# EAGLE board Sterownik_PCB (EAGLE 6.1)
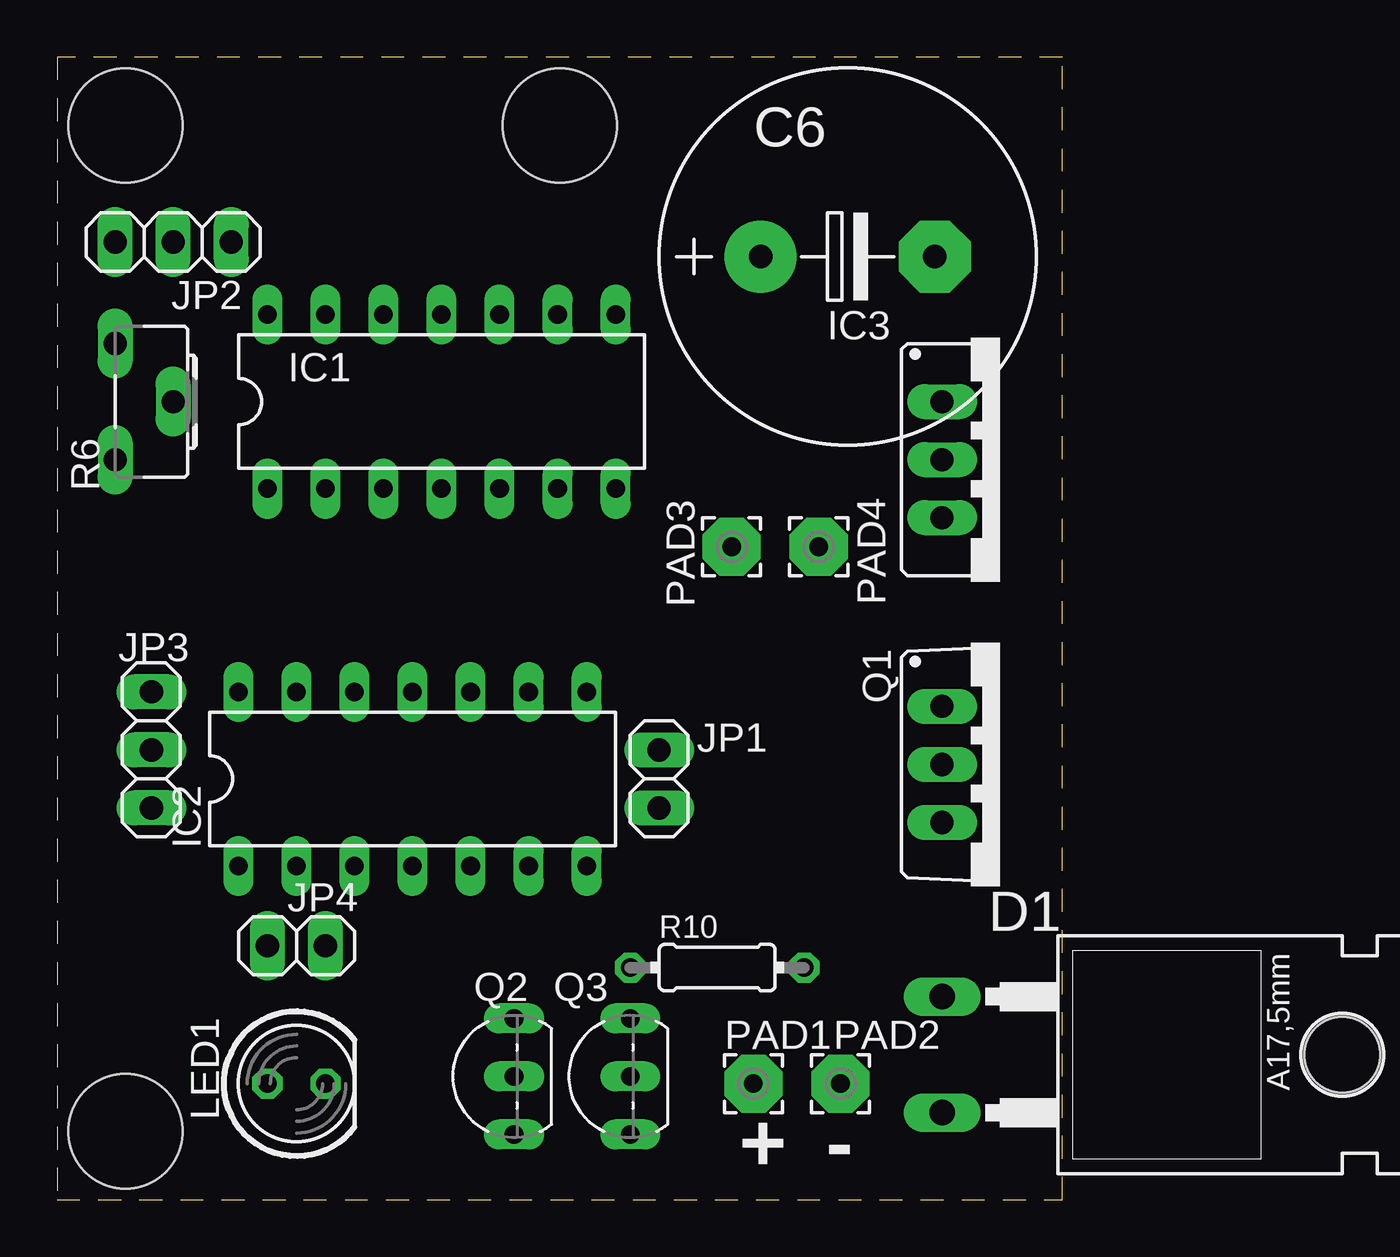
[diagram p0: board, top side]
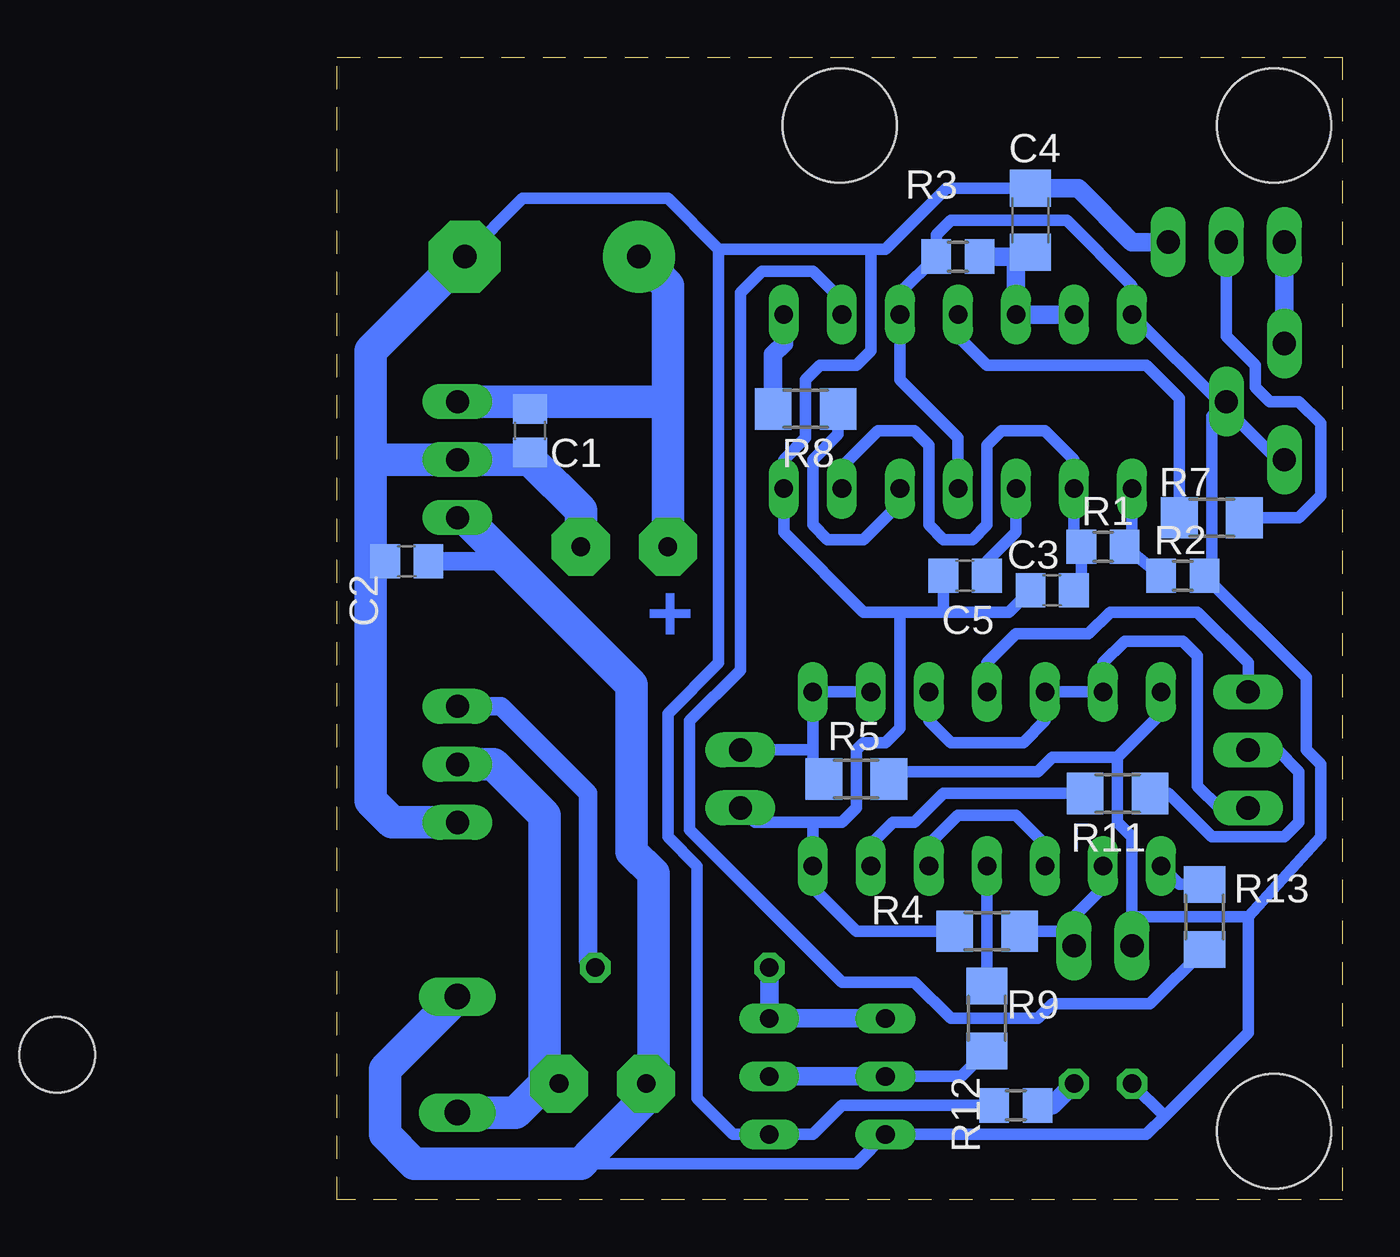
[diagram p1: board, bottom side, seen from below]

Size 44 x 50 mm. Coordinates in mm from the lower left corner, seen from the top.
Outline: 0,0 44,0 44,50 0,50 0,0
Copper layers (1*16): Top 0.035mm / dielectric 1.5mm / Bottom 0.035mm
Design rules: minimum track width 20mil, minimum drill 24mil, track to track 8mil, track to pad 8mil, pad to pad 8mil, via to via 8mil, smd to smd 8mil, copper to edge 10mil, drill to drill 8mil, minimum pad ring 10mil, minimum via ring 8mil, stop-mask expansion 4mil, vias tented up to drill 0mil, thermal gap 10mil
Holes 5 mm at 3,47 3,3 22,47

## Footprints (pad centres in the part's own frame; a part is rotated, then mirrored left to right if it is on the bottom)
C0805 = smd 1.3 x 1.5: 1 -0.95,0; 2 0.95,0
C1206 = smd 1.6 x 1.8: 1 -1.4,0; 2 1.4,0
E7,5-16 = drill 1.016 pad 3.15: + -3.81,0 | drill 1.016 pad 3.15 octagon: - 3.81,0
TO220AC = drill 1.118 long: A 2.54,-6.35; C -2.54,-6.35 | hole 3.302: 0,11.176
DIL14 = drill 0.813 long: 1 -7.62,-3.81; 2 -5.08,-3.81; 3 -2.54,-3.81; 4 0,-3.81; 5 2.54,-3.81; 6 5.08,-3.81; 7 7.62,-3.81; 8 7.62,3.81; 9 5.08,3.81; 10 2.54,3.81; 11 0,3.81; 12 -2.54,3.81; 13 -5.08,3.81; 14 -7.62,3.81
78XXS = drill 1.016 long: GND 0,-2.54; IN -2.54,-2.54; OUT 2.54,-2.54
1X02 = drill 1.016 long: 1 -1.27,0; 2 1.27,0
1X03 = drill 1.016 long: 1 -2.54,0; 2 0,0; 3 2.54,0
LED5MM = drill 0.813 octagon: A -1.27,0; K 1.27,0
2,54/0,8 = drill 0.813 pad 2.54 octagon: 1 0,0
TO220BV = drill 1.016 long: D 0,-2.54; G -2.54,-2.54; S 2.54,-2.54
TO92-EBC = drill 0.813 long: B 0,-1.27; C -2.54,-1.27; E 2.54,-1.27
R0805 = smd 1.3 x 1.5: 1 -0.95,0; 2 0.95,0
R1206 = smd 1.6 x 1.803: 1 -1.422,0; 2 1.422,0
CA6H = drill 1.016 long: A -2.54,0; E 2.54,0; S 0,2.54
0204/7 = drill 0.813 octagon: 1 -3.81,0; 2 3.81,0

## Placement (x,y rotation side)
C1  100n  [C0805]  35.56,33.66 270 bottom
C2  100n  [C0805]  40.96,27.94 180 bottom
C3  100n  [C0805]  12.7,26.67 180 bottom
C4  100n  [C1206]  13.65,42.86 90 bottom
C5  10n  [C0805]  16.51,27.3 180 bottom
C6  4700u  [E7,5-16]  34.61,41.27 0 top
D1  MBR1060  [TO220AC]  45.09,6.35 270 top
IC1  NE556N  [DIL14]  16.83,34.92 0 top
IC2  4093N  [DIL14]  15.56,18.41 0 top
IC3  78S12  [78XXS]  41.27,32.38 270 top
JP1  Switch  [1X02]  26.35,18.41 270 top
JP2  Obroty  [1X03]  5.08,41.91 0 top
JP3  Polaryzacja  [1X03]  4.13,19.68 90 top
JP4  Generator  [1X02]  10.48,11.11 0 top
LED1  G  [LED5MM]  10.48,5.08 0 top
PAD1  [2,54/0,8]  30.48,5.08 0 top
PAD2  [2,54/0,8]  34.29,5.08 0 top
PAD3  [2,54/0,8]  29.53,28.57 0 top
PAD4  [2,54/0,8]  33.34,28.57 0 top
Q1  IRF520  [TO220BV]  41.27,19.05 270 top
Q2  BC546B  [TO92-EBC]  18.73,5.4 90 top
Q3  BC558C  [TO92-EBC]  23.81,5.4 90 top
R1  10k  [R0805]  10.48,28.57 0 bottom
R2  4k7  [R0805]  6.99,27.3 0 bottom
R3  10k  [R0805]  16.83,41.27 180 bottom
R4  10k  [R1206]  15.56,11.75 0 bottom
R5  10k  [R1206]  21.27,18.41 0 bottom
R6  10k  [CA6H]  2.54,34.92 270 top
R7  0  [R1206]  5.71,29.84 180 bottom
R8  0  [R1206]  23.5,34.61 180 bottom
R9  10k  [R1206]  15.56,7.94 270 bottom
R10  33  [0204/7]  28.89,10.16 0 top
R11  0  [R1206]  9.84,17.78 180 bottom
R12  2k2  [R0805]  14.29,4.13 0 bottom
R13  0  [R1206]  6.03,12.38 90 bottom

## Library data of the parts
C1-C6 R1-R5 R7-R13 = rcl
D1 = diode
IC1 = linear
IC2 = 40xx
IC3 = v-reg
JP1-JP4 = pinhead
LED1 = led
PAD1-PAD4 = wirepad
Q1 = transistor-power
Q2 = transistor-npn
Q3 = transistor-pnp
R6 = pot

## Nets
+12V: C2.1 D1.C IC1.4 IC1.10 IC1.14 IC2.14 IC3.OUT JP4.1 LED1.A PAD1.1 Q2.C R2.2 R3.2 R5.2 R6.E R6.S
GND: C1.2 C2.2 C3.2 C4.2 C5.2 C6.- IC1.7 IC2.7 IC3.GND JP1.2 JP2.3 PAD4.1 Q1.S Q3.C R4.1 R12.1
N$1: IC1.5 R8.1
N$2: C5.1 IC1.3
N$3: C3.1 IC1.2 IC1.6 R1.1
N$4: IC1.1 R1.2 R2.1
N$5: C4.1 IC1.12 IC1.13 R3.1
N$6: IC2.2 JP4.2 R4.2
N$7: IC2.1 R13.2
N$8: IC2.8 IC2.9 JP1.1 R5.1
N$9: JP3.2 R11.1
N$10: IC2.10 IC2.12 IC2.13 JP3.1
N$11: IC2.11 JP3.3
N$12: IC2.3 IC2.5
N$13: IC2.4 R9.1
N$14: C1.1 C6.+ IC3.IN PAD3.1
N$15: JP2.1 R6.A
N$16: JP2.2 R7.1
N$17: D1.A PAD2.1 Q1.D
N$18: IC1.11 R7.2
N$19: IC1.8 R8.2
N$20: Q2.B Q3.B R9.2
N$21: Q2.E Q3.E R10.1
N$22: Q1.G R10.2
N$23: IC2.6 R11.2
N$24: LED1.K R12.2
N$25: IC1.9 R13.1

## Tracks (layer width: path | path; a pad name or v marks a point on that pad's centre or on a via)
+12V
  Bottom 0.508: IC1.4 16.83,33.34 19.37,35.88 IC1.10 19.37,39.69 R3.2 17.78,42.23 17.14,42.86 12.06,42.86 9.21,40.01 IC1.14 5.24,34.77 | R6.E 2.86,32.38 5.24,34.77 | R6.S | R6.S 5.24,34.77 | R6.S 5.71,34.29 5.71,27.62 R2.2 1.59,22.86 1.59,19.68 0.95,19.05 0.95,15.88 4.13,12.38 | 9.21,12.38 JP4.1 | 9.21,12.38 9.21,15.88 9.84,16.51 9.84,19.37 | 9.84,19.37 7.94,21.27 IC2.14 | 9.84,19.37 12.7,19.37 13.34,18.73 19.53,18.73 R5.2 | 4.13,12.38 9.21,12.38 | 7.78,3.65 4.13,7.3 4.13,12.38 | 7.78,3.65 8.57,2.86 Q2.C 21.27,1.59 32.7,1.59 33.02,1.91 | LED1.A | 7.78,3.65 LED1.A
  Bottom 0.813: 36.51,27.94 C2.1
  Bottom 1.422: D1.C 41.91,5.71 41.91,2.86 40.64,1.59 33.34,1.59 33.02,1.91 30.16,4.76 30.16,5.08 | 30.16,5.08 30.16,14.29 31.11,15.24 31.11,22.54 36.51,27.94 38.42,29.84 IC3.OUT | 30.16,5.08 PAD1.1
GND
  Bottom 0.508: C3.2 14.6,25.72 17.46,25.72 | C5.2 17.46,25.72 | 20.64,41.59 20.64,37.15 21.27,36.51 22.86,36.51 23.5,35.88 23.5,33.34 24.45,32.38 IC1.7 24.45,29.21 20.95,25.72 19.37,25.72 | R4.1 21.27,11.75 23.18,13.65 IC2.7 23.18,16.51 | 19.37,25.72 17.46,25.72 | 19.37,25.72 19.37,20.64 20,20 20.95,20 21.27,19.68 21.27,17.14 21.91,16.51 23.18,16.51 | 23.18,16.51 25.72,16.51 JP1.2 | C4.2 17.33,44.26 20,41.59 20.64,41.59 | 27.3,41.59 20.64,41.59 | 27.3,41.59 27.3,23.5 29.53,21.27 29.53,15.88 28.26,14.61 28.26,4.45 26.67,2.86 Q3.C 23.18,2.86 21.91,4.13 R12.1 | C6.- 35.88,43.81 29.53,43.81 27.3,41.59 | 35.56,32.38 C1.2 | 42.55,27.94 C2.2
  Bottom 0.813: C4.2 11.56,44.26 9.21,41.91 JP2.3
  Bottom 1.422: Q1.S 41.59,16.51 42.55,17.46 42.55,27.94 42.55,32.38 | 42.55,32.38 IC3.GND 35.56,32.38 33.34,30.16 PAD4.1 | 42.55,32.38 42.55,37.15 C6.-
N$1
  Bottom 0.508: IC1.5 19.37,30.48 20.95,28.89 22.54,28.89 23.18,29.53 23.18,32.38 22.07,33.49 R8.1
N$2
  Bottom 0.508: C5.1 15.56,27.94 14.29,29.21 IC1.3
N$3
  Bottom 0.508: IC1.6 21.91,32.07 20.32,33.66 18.73,33.66 18.1,33.02 18.1,29.53 17.46,28.89 16.19,28.89 15.56,29.53 15.56,33.02 14.92,33.66 13.02,33.66 11.75,32.38 IC1.2 11.75,28.89 R1.1 11.43,26.99 C3.1
N$4
  Bottom 0.508: R2.1 R1.2 9.21,28.89 IC1.1
N$5
  Bottom 0.813: IC1.13 IC1.12 14.29,41.27 | 14.29,41.27 13.84,41.27 C4.1 | 14.29,41.27 R3.1
N$6
  Bottom 0.508: IC2.2 10.48,13.65 11.75,12.38 11.75,11.75 | JP4.2 11.75,11.75 | 11.75,11.75 R4.2
N$7
  Bottom 0.508: R13.2 7.14,13.8 IC2.1
N$8
  Bottom 0.508: IC2.9 IC2.8 23.18,19.68 | 23.18,19.68 23.18,19.21 R5.1 | 23.18,19.68 JP1.1
N$9
  Bottom 0.508: R11.1 7.62,17.78 5.71,15.88 2.54,15.88 1.91,16.51 1.91,18.73 2.86,19.68 JP3.2
N$10
  Bottom 0.508: IC2.10 18.1,20.95 17.14,20 13.97,20 13.02,20.95 IC2.12 IC2.13 10.48,23.5 9.53,24.45 6.99,24.45 6.35,23.81 6.35,18.1 5.4,17.14 JP3.1
N$11
  Bottom 0.508: IC2.11 15.56,23.5 14.29,24.77 11.11,24.77 10.16,25.72 6.35,25.72 4.13,23.5 JP3.3
N$12
  Bottom 0.508: IC2.3 13.02,15.56 14.29,16.83 16.83,16.83 18.1,15.56 IC2.5
N$13
  Bottom 0.508: R9.1 IC2.4
N$14
  Bottom 0.508: 35.88,34.92 C1.1
  Bottom 1.422: PAD3.1 29.53,34.92 | 29.53,34.92 29.53,40.01 C6.+ | 29.53,34.92 35.88,34.92 IC3.IN
N$15
  Bottom 0.813: R6.A JP2.1
N$16
  Bottom 0.508: JP2.2 5.08,37.78 3.81,36.51 3.81,35.56 3.17,34.92 1.91,34.92 0.95,33.97 0.95,30.8 1.91,29.84 R7.1
N$17
  Bottom 1.422: Q1.D 37.15,19.05 34.92,16.83 34.92,5.08 | D1.A 36.2,3.81 34.92,5.08 | PAD2.1 34.92,5.08
N$18
  Bottom 0.508: R7.2 7.14,35.08 8.57,36.51 15.56,36.51 16.83,37.78 IC1.11
N$19
  Bottom 0.813: R8.2 24.92,36.99 24.45,37.47 IC1.8
N$20
  Bottom 0.508: Q2.B 16.68,5.4 R9.2
  Bottom 0.813: Q2.B Q3.B
N$21
  Bottom 0.813: R10.1 Q3.E Q2.E
N$22
  Bottom 0.813: Q1.G 36.83,21.59 33.02,17.78 33.02,10.48 R10.2
N$23
  Bottom 0.508: R11.2 17.46,17.78 18.73,16.51 19.68,16.51 20.64,15.56 IC2.6
N$24
  Bottom 0.813: R12.2 12.7,4.13 LED1.K
N$25
  Bottom 0.508: IC1.9 21.91,39.37 23.18,40.64 25.4,40.64 26.35,39.69 26.35,23.18 28.57,20.95 28.57,16.19 21.91,9.53 18.73,9.53 17.14,7.94 13.34,7.94 12.7,8.57 8.42,8.57 R13.1

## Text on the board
Bottom: +
tPlace: + | -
